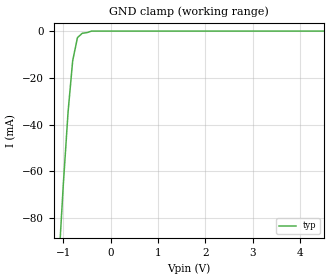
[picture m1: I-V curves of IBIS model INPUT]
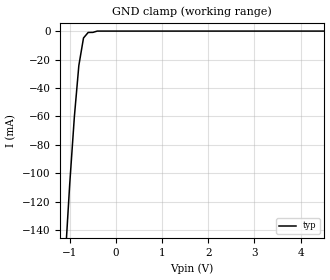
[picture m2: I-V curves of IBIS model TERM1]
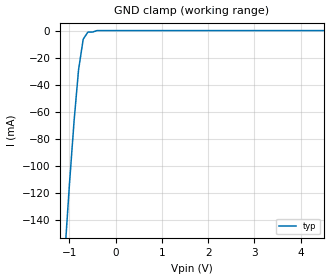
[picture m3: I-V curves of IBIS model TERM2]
|   PERICOM SEMICONDUCTOR CORP
|   IBIS Model of PI5A3157
|   Product Family: 5A
|   UDFN (ZU) Package
[IBIS Ver] 3.2
[Comment char] |_char
[File Name] pi5a3157b_zu_33v.ibs
[File Rev] 2.1
[Source] File originated at Pericom Semiconductor Corp.
[Date] 07/28/17
[Disclaimer] (C) Copyright PERICOM Semiconductor Corporation
   All rights reserved
  Pericom Semiconductor Corporation hereby grants the user of
  this IBIS model a non-exclusive, nontransferable license to
  use this IBIS model under the following terms.
  This IBIS model is provided on an "AS IS" basis and Pericom
  makes absolutely no warranty with respect to the information
  contained herein. PERICOM DISCLAIMS AND CUSTOMER WAIVES ALL
  WARRANTIES, EXPRESSED OR IMPLIED, INCLUDING WARRANTIES OF
  MERCHANTABILITY OR FITNESS FOR A PARTICULAR PURPOSE. The
  entire risk as to quality and performance is with the customer.
  Accordingly, in no event shall the company be liable for any
  damages, whether in contract or tort, including any lost
  profits or other incidental, consequential, exemplary, or
  punitive damages arising out of the use or application of the
  IBIS model provided in this package. Further, Pericom reserves
  the right to make changes without notice to any product herein
  to improve reliability, function, or design. Pericom does not
  convey any license under patent rights or any other intellectual
  property rights, including those of third parties.
  The user is granted this license only to use the IBIS model
  and is not granted rights to sell, load, rent, lease or license
  the IBIS model in whole or in part, or in modified form to anyone
  other than user. User may modify the IBIS model to suit its specific
  application but rights to derivative works and such modifications
  shall belong to Pericom.
  Pericom is not obligated to provide maintenance or support
  for the licensed IBIS model.
  Contact Pericom at ATTN: APPLICATION ENGINEERING / IBIS MODELS
  1545 Barber Lane Milpitas, CA 95035 USA.
[Component] PI5A3157B
[Manufacturer] Pericom Semiconductor Corp.
[Package]
| variable   typ   min  max
R_pkg   0.02242ohm   NA   NA
L_pkg   0.95600nH   NA   NA
C_pkg   0.16170pF   NA   NA
[Pin] signal_name   model_name   R_pin   L_pin   C_pin
1   VCC   POWER   0.02320   0.99800nH   0.14900pF
2   B1   TERM1   0.02085   0.87200nH   0.18710pF
3   A   TERM2   0.02320   0.99800nH   0.14900pF
4   B0   TERM1   0.02320   0.99800nH   0.14900pF
5   GND   GND   0.02085   0.87200nH   0.18710pF
6   S   INPUT   0.02320   0.99800nH   0.14900pF
[Series Switch Groups]
On 1 /
Off 2 /
[Series Pin Mapping]   pin_2   model_name  function_table_group
3   4   SWITCH1   1
3   2   SWITCH1   2
|   Model SWITCH1
[Model] SWITCH1
Model_type Series_switch
| variable   typ   min   max
C_comp   18.5000pF  NA   NA
[Voltage Range]   3.3000V   NA   NA
[POWER Clamp Reference]   3.3000V   NA   NA
[GND Clamp Reference]   0.0000V   NA   NA
[On]
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[OFF]
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| Models and submodels in the file (4): INPUT (Input), SWITCH1 (Series_switch), TERM1 (Terminator), TERM2 (Terminator)
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|   Model INPUT
[Model] INPUT
Model_type Input
Vinl = 825mV
Vinh = 2.310V
| variable   typ   min   max
C_comp   2.3000pF   NA   NA
[Voltage Range]   3.3000V   NA   NA
[GND Clamp Reference]   0.0000V   NA   NA
[POWER Clamp Reference]   3.3000V   NA   NA
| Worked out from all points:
|   GND clamp passes 1 mA (typ) near -0.60 V on its own axis
[GND Clamp]
| Voltage   I(typ)   I(min)   I(max)
-3.3V     -906.3mA   NA         NA
-1.1V     -101mA     NA         NA
-999.3mV  -65.49mA   NA         NA
-898.2mV  -34.4mA    NA         NA
-802mV    -12.71mA   NA         NA
-700.9mV  -2.78mA    NA         NA
-599.7mV  -950uA     NA         NA
-402.6mV  0A         NA         NA
6.602V    0A         NA         NA
[POWER Clamp]   |Note: Vtable = Vcc - Voutput
| Voltage   I(typ)   I(min)   I(max)
-3.3V     0A         NA         NA
0V        0A         NA         NA
|   Model TERM1
[Model] TERM1
Model_type Terminator
| variable   typ   min   max
C_comp   6.5000pF   NA   NA
[Voltage Range]   3.3000V   NA   NA
[GND Clamp Reference]   0.0000V   NA   NA
[POWER Clamp Reference]   3.3000V   NA   NA
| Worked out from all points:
|   GND clamp passes 1 mA (typ) near -0.60 V on its own axis
[GND Clamp]
| Voltage   I(typ)   I(min)  I(max)
-3.3V     -1.236A    NA         NA
-1.1V     -162.2mA   NA         NA
-999.3mV  -107.7mA   NA         NA
-898.2mV  -60.09mA   NA         NA
-802mV    -24.25mA   NA         NA
-700.8mV  -4.84mA    NA         NA
-599.7mV  -960uA     NA         NA
-498.4mV  -920uA     NA         NA
-402.6mV  0A         NA         NA
6.602V    0A         NA         NA
[POWER Clamp]   |Note: Vtable = Vcc - Voutput
| Voltage   I(typ)   I(min)   I(max)
-3.3V     0A         NA         NA
0V        0A         NA         NA
|   Model TERM2
[Model] TERM2
Model_type Terminator
| variable   typ   min   max
C_comp   11.5000pF   NA   NA
[Voltage Range]   3.3000V   NA   NA
[GND Clamp Reference]   0.0000V   NA   NA
[POWER Clamp Reference]   3.3000V   NA   NA
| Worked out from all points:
|   GND clamp passes 1 mA (typ) near -0.49 V on its own axis
[GND Clamp]
| Voltage   I(typ)   I(min)  I(max)
-3.3V     -1.118A    NA         NA
-1.1V     -165.5mA   NA         NA
-999.3mV  -113.4mA   NA         NA
-898.2mV  -66.37mA   NA         NA
-802mV    -28.86mA   NA         NA
-700.8mV  -6.27mA    NA         NA
-599.7mV  -1.13mA    NA         NA
-498.4mV  -1.09mA    NA         NA
-402.6mV  0A         NA         NA
6.602V    0A         NA         NA
[POWER Clamp]   |Note: Vtable = Vcc - Voutput
| Voltage   I(typ)   I(min)   I(max)
-3.3V     0A         NA         NA
0V        0A         NA         NA
